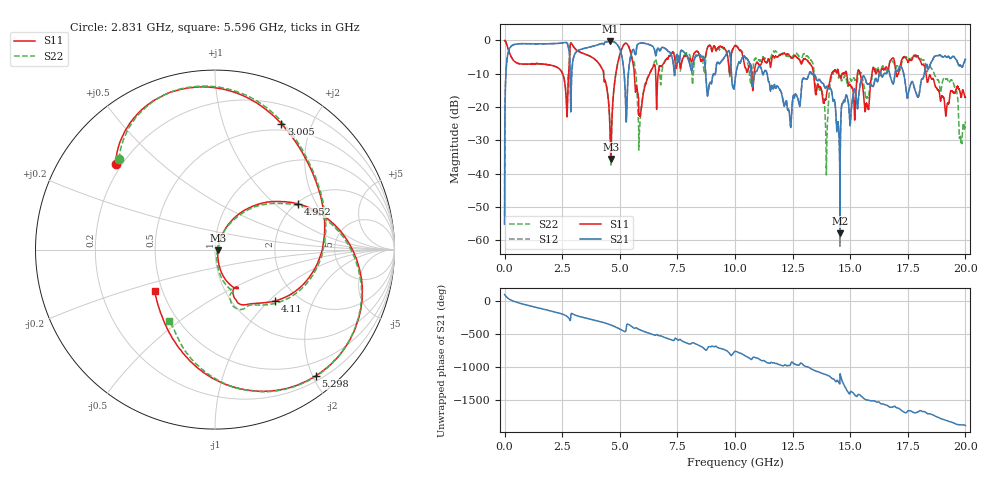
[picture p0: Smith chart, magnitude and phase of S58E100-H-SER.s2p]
!{S58E100}
!Johanson Technology Inc.
!www.johansontechnology.com
!Test Board Conditions:
!Substrate Type  RO4350B
!Substrate Thickness  60 mil
!Substrate Dk  3.66
!TL Type: GCPW
!TL Trace Width  115 mil
!TL Gap  52 mil
!Electrode orientation  Horizontal
!DUT TOPOLOGY	SERIES
!Mounting Pad LxW  55x428 mil
! Created Tue Apr 13 22:44:27 2021
# mhz S ma R 50
! 2 Port Network Data from SP1.SP block
! freq  magS11  angS11  magS21  angS21  magS12  angS12  magS22  angS22
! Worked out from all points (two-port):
!   20001 points, 300 kHz to 20 GHz, reference 50 ohm
!   highest |S21| = -0.24 dB at 4.59 GHz (marker M1); lowest = -57.9 dB at 14.56 GHz (marker M2)
!   |S21| within 3 dB of the highest: 173.5 MHz to 2.806 GHz (2.633 GHz wide, 177 % of centre); 3.144 GHz to 5.032 GHz (1.889 GHz wide, 46.2 % of centre)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
!   lowest |S11| = -35.5 dB at 4.61 GHz (marker M3), VSWR 1.03, Z = 51.7 - j0.394 ohm
!   |S11| at or under -10 dB: 5.629 GHz to 6.296 GHz (666.4 MHz wide, 11.2 % of centre); 13.41 GHz to 14.2 GHz (785.2 MHz wide, 5.69 % of centre); 18.29 GHz to end of sweep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
!   |S22| runs from -40.3 to 0.0 dB; largest |S21 - S12| = 0.012
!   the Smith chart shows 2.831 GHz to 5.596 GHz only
!   S11 on the Smith chart (normalised r, x): 2.831 GHz: 0.18, +0.36; 3.005 GHz: 0.42, +1.58; 4.11 GHz: 1.54, -1.09; 4.952 GHz: 2.04, +1.44; 5.298 GHz: 0.28, -2.05; 5.596 GHz: 0.45, -0.25
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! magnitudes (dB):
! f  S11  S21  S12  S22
! 300 kHz  -0.1  -55.2  -55.2  -0.1
! 108.3 MHz  -1.5  -5.5  -5.5  -1.5
! 276.3 MHz  -4.8  -1.8  -1.8  -4.7
! 2.831 GHz  -2.7  -6.4  -6.4  -2.7
! 3.005 GHz  -2.0  -4.8  -4.8  -2.0
! 3.334 GHz  -3.7  -2.6  -2.6  -3.7
! 4.11 GHz  -7.1  -1.2  -1.2  -7.1
! 4.59 GHz  -30.0  -0.2  -0.3  -30.2
! 4.61 GHz  -35.5  -0.3  -0.3  -37.0
! 4.952 GHz  -5.6  -1.9  -1.9  -5.6
! 5.298 GHz  -0.9  -21.2  -21.1  -0.9
! 5.596 GHz  -7.8  -2.7  -2.7  -6.5
! 5.864 GHz  -22.7  -0.9  -0.9  -25.8
! 6.667 GHz  -9.8  -2.3  -2.3  -7.8
! 10 GHz  -1.5  -11.9  -11.9  -1.7
! 12.37 GHz  -4.6  -22.5  -22.1  -5.0
! 13.33 GHz  -7.7  -10.0  -10.0  -6.2
! 13.96 GHz  -17.0  -13.9  -13.8  -37.3
! 14.56 GHz  -10.7  -57.9  -61.7  -10.3
! 15.72 GHz  -19.0  -12.9  -12.8  -17.0
! 16.67 GHz  -8.6  -8.9  -8.9  -8.1
! 20 GHz  -17.1  -5.6  -5.5  -24.3
